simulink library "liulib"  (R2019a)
settings: Solver=ode45  StartTime=0.0  StopTime=10.0  RelTol=1e-3  EnableMultiTasking=on
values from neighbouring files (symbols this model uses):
  ag = NaN(L.ng,1)    [bdet.m]
  D = meqp()    [fbtp.m]
  dr2FA = dr2Fs(1:nA,1)    [asxycs.m]
  drzFA = drzFs(1:nA,1)    [asxycs.m]
  dz = dzxs(is)    [asxycsJac.m]    (also in bintc.m = (z - zx(kz))/dzx)
  dz2FA = dz2Fs(1:nA,1)    [asxycs.m]
  err = [IaeH            ; IoeH               ; IueH               ; DeH               ; FeH            ; BeH               ; BeH               ; BeH               ; CeH               ; CeH               ; CeH               ; VeH                ; VeH                ; VeH               ]    [fbtopt.m]
  FA = Fs(1:nA,1)    [asxycs.m]    (also in bfhelp.m = [-1                        0        0       ])
  FB = [0                         1        1       ]    [bfhelp.m]
  Fx = meqFx(L,Iy,[Ia;Iu])    [bdet.m]    (also in bfhelp.m = zeros(n+2,3); Fx(2:end-1,2) = FN)
  FX = Fs(nA+1:ns,1)    [asxycs.m]
  IpD = LXs.Ip    [fbtinit.m]
  Iy = LXt.Iy    [bdet.m]    (also in fbtinit.m = meqinitIy(L,LXs.t,IpD,bbs,LXs.capaj))
  L = fbtc(P,G)    [fbt.m]    (also in fbtc.m = meqc(P,G); fbte.m = varargout{1})
  nA = numel(rA)    [asxycs.m]
  niter = L.P.itercs    [asxycs.m]
  Opy = logical(Opy)    [bfct.m]    (also in bfdoublet.m = Opy==1 | Opy==2)
  rA = rs(1:nA,1)    [asxycs.m]    (also in fbtptcv.m = (rA1 + 3*rA2)/4)
  rX = rs(nA+1:ns,1)    [asxycs.m]    (also in fbtptcv.m = rzbro(iX,1); fbtxana.m = r0)
  zA = zs(1:nA,1)    [asxycs.m]    (also in fbtptcv.m = (zA1 + 3*zA2)/4)
  zX = zs(nA+1:ns,1)    [asxycs.m]    (also in fbtptcv.m = rzbro(iX,2); fbtxana.m = 0)
undefined symbols (not defined in the file or in its folder): aminor, aq, aW, Bm, bp, bpli2, Brn, Brrn, Brzn, bt, Bzn, Bzrn, Bzzn, delta, deltal, deltau, dzg, epsilon, Ff, Fn, Ft, Ft0, FW, Ie, Ip, iqQ, iTQ, jtorQ, kappa, lB, li, lp, lX, mu, nX, PpQ, PQ, Q0Q, Q1Q, Q2Q, Q3Q, Q4Q, q95, qmin, raQ, raqmin, rB, rbary, rBt, repmat, rgeom, rIp, rIpD, Row, rq, rS, rst, rYD, TQ, TTpQ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
libraries: $bdroot x53, mkllib x48, simulink x7
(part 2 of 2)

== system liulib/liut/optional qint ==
  "LY " : Inport
  Fx : Inport  Port=2
  direct pass : Subsystem  VariantControl=liuINFCTMODEvariant1
  "qint " : Subsystem  VariantControl=liuINFCTMODEvariant2
  " LYo" : Outport

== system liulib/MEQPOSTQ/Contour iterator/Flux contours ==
  zaq : Inport
  rst : Inport  Port=2
  rA : Inport  Port=3
  zA : Inport  Port=4
  FA : Inport  Port=5
  FB : Inport  Port=6
  Fx : Inport  Port=7
  Opy : Inport  Port=8
  IC=1 : UnitDelay  InitialCondition=1  SampleTime=-1  HasFrameUpgradeWarning=on
  Opo : Constant  Value=int8(1)
  RTCI : $bdroot/RTCI  c=L.cdrq  s=L.cdzq  da=L.drx  nr=L.nrx  nz=L.nzx
  Sum : Sum  Inputs=|+-
  Sum1 : Sum  Inputs=|+-
  Sum5 : Sum  Inputs=|+-
  "aq " : Switch  Criteria=u2 ~= 0
  aq0 : Subsystem  TreatAsAtomicUnit=on
  dan : Terminator
  fq : Gain  Gain=L.fq  ParamDataTypeStr=single  OutDataTypeStr=single
  idrx : Gain  Gain=L.idrx  ParamDataTypeStr=single  OutDataTypeStr=single
  idzx : Gain  Gain=L.idzx  ParamDataTypeStr=single  OutDataTypeStr=single
  qaq3 : Sum  Inputs=|++
  rx1 : Constant  Value=L.G.rx(1)  OutDataTypeStr=single
  zx1 : Constant  Value=L.G.zx(1)  OutDataTypeStr=single
  aq : Outport
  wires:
  qaq3/1 -> RTCI/5
  Fx/1 -> RTCI/4
  idzx/1 -> RTCI/3
  idrx/1 -> RTCI/2
  RTCI/2 -> dan/1
  zaq/1 -> "aq "/3
  aq0/1(aq) -> "aq "/1
  "aq "/1 -> RTCI/1
  rA/1 -> Sum/1, aq0/1(rA)
  rx1/1 -> Sum/2
  Sum/1 -> idrx/1
  zA/1 -> Sum1/1, aq0/2(zA)
  zx1/1 -> Sum1/2
  Sum1/1 -> idzx/1
  Sum5/1 -> fq/1
  fq/1 -> qaq3/1
  FB/1 -> Sum5/2, qaq3/2
  FA/1 -> RTCI/7, Sum5/1
  RTCI/1 -> aq/1  "aq"
  Opy/1 -> RTCI/6
  Opo/1 -> RTCI/8
  rst/1 -> IC=1/1
  IC=1/1 -> aq0/Enable, "aq "/2

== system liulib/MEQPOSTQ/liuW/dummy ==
  LY : Inport
  LYo : Outport
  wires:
  LY/1 -> LYo/1

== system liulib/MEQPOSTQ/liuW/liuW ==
  LY : Inport
  Bus Assignment : BusAssignment  AssignedSignals=aW,FW
  Bus Selector : BusSelector  OutputSignals=rst,Fx,Opy,FB,FX,lX,nX
  MATLAB Function : MATLAB Function  TreatAsAtomicUnit=on  mask{nFW=L.P.nFW}
  liuW : Subsystem  VariantControl=liuAWMODEvariant1
  LYo : Outport
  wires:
  Bus Selector/7 -> MATLAB Function/4(nX)  "<nX>"
  Bus Selector/6 -> MATLAB Function/3(lX)  "<lX>"
  Bus Selector/5 -> MATLAB Function/2(FX)  "<FX>"
  Bus Selector/4 -> MATLAB Function/1(FB)  "<FB>"
  Bus Selector/2 -> liuW/2(Fx)  "<Fx>"
  Bus Selector/3 -> liuW/3(Opy)  "<Opy>"
  Bus Selector/1 -> liuW/1(rst)  "<rst>"
  LY/1 -> Bus Selector/1, Bus Assignment/1
  MATLAB Function/1(FW) -> Bus Assignment/3, liuW/4(FW)
  liuW/1(aW) -> Bus Assignment/2
  Bus Assignment/1 -> LYo/1

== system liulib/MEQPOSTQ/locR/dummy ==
  LY : Inport
  "raQ " : Inport  Port=2
  "qQ " : Inport  Port=3
  sq : Inport  Port=4
  Terminator : Terminator
  Terminator1 : Terminator
  Terminator2 : Terminator
  " LYo" : Outport
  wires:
  "raQ "/1 -> Terminator/1
  "qQ "/1 -> Terminator1/1
  sq/1 -> Terminator2/1
  LY/1 -> " LYo"/1

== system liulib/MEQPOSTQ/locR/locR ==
  LY : Inport
  raQ : Inport  Port=2
  qQ : Inport  Port=3
  sq : Inport  Port=4
  Apply sign : Product  Inputs=**
  Bus Assignment : BusAssignment  AssignedSignals=raR
  Constant3 : Constant  Value=L.P.iqR  OutDataTypeStr=single
  Constant4 : Constant  Value=L.raN  OutDataTypeStr=single
  locR : $bdroot/locR  nR=L.nR  naR=L.P.naR
  " LYo" : Outport
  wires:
  Constant4/1 -> locR/4
  qQ/1 -> locR/2
  sq/1 -> Apply sign/2
  Apply sign/1 -> locR/3
  raQ/1 -> locR/1
  Constant3/1 -> Apply sign/1
  locR/1 -> Bus Assignment/2  "raR"
  LY/1 -> Bus Assignment/1
  Bus Assignment/1 -> " LYo"/1

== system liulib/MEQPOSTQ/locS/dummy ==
  "LY " : Inport
  " LYo" : Outport
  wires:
  "LY "/1 -> " LYo"/1

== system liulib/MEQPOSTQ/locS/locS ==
  LY : Inport
  Bus Assignment4 : BusAssignment  AssignedSignals=rS,zS
  Bus Selector : BusSelector  OutputSignals=aq,raQ,rA,zA
  Constant1 : Constant  Value=L.P.raS  OutDataTypeStr=single
  Constant2 : Constant  Value=L.raN  OutDataTypeStr=single
  Matrix Concatenate : Concatenate  Mode=Multidimensional array  ConcatenateDimension=2
  RTCI1 : $bdroot/RTCI1  SFunctionModules=''
  RTCI2 : $bdroot/RTCI1  SFunctionModules=''
  crq : Constant  Value=L.crq  OutDataTypeStr=single
  czq : Constant  Value=L.czq  OutDataTypeStr=single
  locS : $bdroot/locS  SFunctionModules=''
  row of zeros : Constant  Value=zeros(L.noq,1)  OutDataTypeStr=Inherit: Inherit via back propagation
  LYo : Outport
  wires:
  Bus Selector/4 -> RTCI2/3  "<zA>"
  Bus Assignment4/1 -> LYo/1
  LY/1 -> Bus Selector/1, Bus Assignment4/1
  locS/1 -> RTCI1/1, RTCI2/1
  Matrix Concatenate/1 -> locS/1
  Bus Selector/2 -> locS/2  "<raQ>"
  Constant1/1 -> locS/3
  czq/1 -> RTCI2/2
  crq/1 -> RTCI1/2
  Bus Selector/3 -> RTCI1/3  "<rA>"
  RTCI2/1 -> Bus Assignment4/3
  RTCI1/1 -> Bus Assignment4/2
  Constant2/1 -> locS/4
  row of zeros/1 -> Matrix Concatenate/1
  Bus Selector/1 -> Matrix Concatenate/2  "<aq>"

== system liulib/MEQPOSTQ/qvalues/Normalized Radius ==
  aq : Inport
  Constant : Constant  Value=0  OutDataTypeStr=single
  Normalise : Product  Inputs=*/
  Outboard radius : Selector  NumberOfDimensions=2  InputPortWidth=3  IndexOptions=Index vector (dialog),Select all  Indices=find(L.crq==1),L.npq  OutputSizes=1,1
  Permute Dimensions : PermuteDimensions
  Reshape : Reshape
  Reshape1 : Reshape
  Vector Concatenate : Concatenate
  end value : Selector  InputPortWidth=L.npq  IndexOptions=Index vector (dialog)  Indices=L.npq  OutputSizes=1
  raQ : Outport
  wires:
  Outboard radius/1 -> Reshape1/1
  Reshape1/1 -> end value/1, Normalise/1
  Constant/1 -> Vector Concatenate/1
  aq/1 -> Outboard radius/1
  Normalise/1 -> Vector Concatenate/2
  end value/1 -> Normalise/2
  Reshape/1 -> raQ/1
  Permute Dimensions/1 -> Reshape/1
  Vector Concatenate/1 -> Permute Dimensions/1

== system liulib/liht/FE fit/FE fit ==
  Yd : Inport
  Ie : Inport  Port=2
  Ip_in : Inport  Port=3
  sIp : Inport  Port=4
  FE : $bdroot/FE  SystemSampleTime=-1  Latency=0  AutoFrameSizeCalculation=off
  Iph : mkllib/A*u  A=L.Iph
  Iph_D : mkllib/A*u  A=[L.Iph_t;L.Iph_b]
  Iprh : mkllib/A*u  A=L.Iprh
  Iprh_D : mkllib/A*u  A=[L.Iprh_t;L.Iprh_b]
  Ipzh : mkllib/A*u  A=L.Ipzh
  Ipzh_D : mkllib/A*u  A=[L.Ipzh_t;L.Ipzh_b]
  Subsystem1 : Subsystem
  Variant Source : VariantSource
  Variant Source1 : VariantSource
  Variant Source2 : VariantSource
  Je : Outport
  IpD : Outport  Port=2
  rIpD : Outport  Port=3
  zIpD : Outport  Port=4
  Ip : Outport  Port=5
  rIp : Outport  Port=6
  zIp : Outport  Port=7
  rYD : Outport  Port=8
  zYD : Outport  Port=9
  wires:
  Variant Source2/1 -> zIpD/1, Subsystem1/3(zIpD)
  Variant Source1/1 -> Subsystem1/2(rIpD), rIpD/1  "rIpD"
  Variant Source/1 -> IpD/1, Subsystem1/1(IpD)
  Subsystem1/1(rYD) -> rYD/1  "rYD"
  Subsystem1/2(zYD) -> zYD/1  "zYD"
  FE/2 -> Je/1
  sIp/1 -> FE/4
  Yd/1 -> FE/1
  Ip_in/1 -> FE/3
  Ie/1 -> FE/2
  Iprh_D/1 -> Variant Source1/1  "rIpD"
  FE/1 -> Iph_D/1, Ipzh/1, Iprh/1, Iph/1, Ipzh_D/1, Iprh_D/1
  Iph_D/1 -> Variant Source/1  "IpD"
  Ipzh_D/1 -> Variant Source2/1  "zIpD"
  Iprh/1 -> rIp/1, Variant Source1/2  "rIp"
  Iph/1 -> Ip/1, Variant Source/2  "Ip"
  Ipzh/1 -> zIp/1, Variant Source2/2  "zIp"

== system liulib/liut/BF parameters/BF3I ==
  BF3I parameters : Subsystem
  Bus Creator : BusCreator  Inputs=4
  bfp : Outport
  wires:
  BF3I parameters/2(IgNg) -> Bus Creator/2
  BF3I parameters/4(fTg) -> Bus Creator/4
  BF3I parameters/3(fPg) -> Bus Creator/3
  Bus Creator/1 -> bfp/1
  BF3I parameters/1(gNg) -> Bus Creator/1

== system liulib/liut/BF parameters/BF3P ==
  Constant : Constant  Value=L.P.bfp
  bfp : Outport
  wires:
  Constant/1 -> bfp/1

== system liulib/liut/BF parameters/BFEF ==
  Constant : Constant  Value=L.P.bfp
  bfp : Outport
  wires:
  Constant/1 -> bfp/1

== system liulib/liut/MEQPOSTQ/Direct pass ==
  "LY " : Inport
  "sIp " : Inport  Port=2
  Terminator : Terminator
  " LYo" : Outport
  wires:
  "LY "/1 -> " LYo"/1
  "sIp "/1 -> Terminator/1

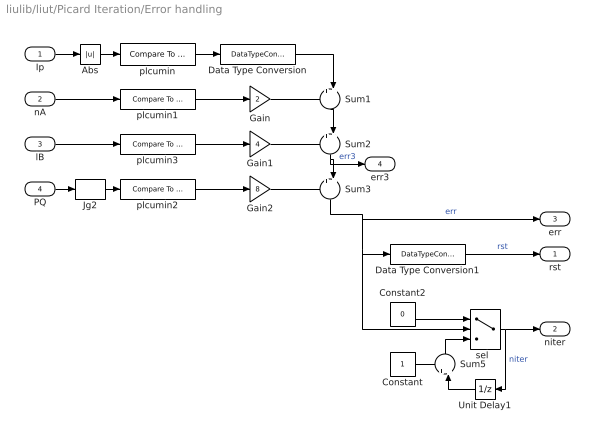
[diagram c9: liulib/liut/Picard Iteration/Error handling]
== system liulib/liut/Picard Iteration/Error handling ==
  Ip : Inport
  nA : Inport  Port=2
  lB : Inport  Port=3
  PQ : Inport  Port=4
  Abs : Abs
  Constant : Constant  VectorParams1D=off  OutDataTypeStr=int32
  Constant2 : Constant  Value=0  VectorParams1D=off  OutDataTypeStr=int32
  Data Type Conversion : DataTypeConversion  OutDataTypeStr=int32
  Data Type Conversion1 : DataTypeConversion  OutDataTypeStr=boolean
  Gain : Gain  Gain=2  OutDataTypeStr=int32
  Gain1 : Gain  Gain=4  OutDataTypeStr=int32
  Gain2 : Gain  Gain=8  OutDataTypeStr=int32
  Jg2 : Selector  IndexMode=Zero-based  IndexOptions=Index vector (dialog)  Indices=0  OutputSizes=1
  Sum{1..3,5} (4 alike) : Sum  Inputs=++|
  Unit Delay1 : UnitDelay  InitialCondition=int32(0)  SampleTime=-1  HasFrameUpgradeWarning=on
  plcumin : simulink/Logic and Bit Operations/Compare To Constant  relop=<  const=L.P.Ipmin  OutDataTypeStr=uint8
  plcumin1 : simulink/Logic and Bit Operations/Compare To Constant  relop===  const=0  OutDataTypeStr=uint8
  plcumin2 : simulink/Logic and Bit Operations/Compare To Constant  relop=<  const=0  OutDataTypeStr=uint8
  plcumin3 : simulink/Logic and Bit Operations/Compare To Constant  relop===  const=0  OutDataTypeStr=uint8
  "sel  " : Switch  Criteria=u2 ~= 0  OutDataTypeStr=int32
  rst : Outport
  niter : Outport  Port=2
  err : Outport  Port=3
  err3 : Outport  Port=4
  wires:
  plcumin2/1 -> Gain2/1
  nA/1 -> plcumin1/1
  Jg2/1 -> plcumin2/1
  PQ/1 -> Jg2/1
  Data Type Conversion1/1 -> rst/1  "rst"
  Ip/1 -> Abs/1
  Abs/1 -> plcumin/1
  "sel  "/1 -> niter/1, Unit Delay1/1  "niter"
  Sum5/1 -> "sel  "/3
  Constant/1 -> Sum5/1
  lB/1 -> plcumin3/1
  plcumin3/1 -> Gain1/1
  Unit Delay1/1 -> Sum5/2
  Constant2/1 -> "sel  "/1
  plcumin1/1 -> Gain/1
  plcumin/1 -> Data Type Conversion/1
  Gain1/1 -> Sum2/1
  Gain2/1 -> Sum3/1
  Sum3/1 -> "sel  "/2, Data Type Conversion1/1, err/1  "err"
  Gain/1 -> Sum1/1
  Data Type Conversion/1 -> Sum1/2
  Sum1/1 -> Sum2/2
  Sum2/1 -> err3/1, Sum3/2  "err3"

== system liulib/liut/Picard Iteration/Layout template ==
  u : Inport
  y : Outport
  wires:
  u/1 -> y/1

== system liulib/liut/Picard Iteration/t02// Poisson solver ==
  rst : Inport
  Yd : Inport  Port=2
  Ie : Inport  Port=3
  Ip : Inport  Port=4
  sIp : Inport  Port=5
  zJy : Inport  Port=6
  zJe : Inport  Port=7
  zdz : Inport  Port=8
  *idzx : Gain  Gain=single(L.idzx)
  Constant2 : Constant  Value=0  OutDataTypeStr=single
  Fb : Switch  Criteria=u2 ~= 0
  Fb BF : Subsystem  TreatAsAtomicUnit=on
  Fb FE : Subsystem  TreatAsAtomicUnit=on
  GSZR : $bdroot/GSZR  cx=L.cx  cq=L.cq  cr=L.cr  cs=L.cs  ci=L.ci  co=L.co
  Je : Switch  Criteria=u2 ~= 0
  Jw : $bdroot/ASGN  iu=L.kyw-1
  "Jy " : Switch  Criteria=u2 ~= 0
  KYWMODE : VariantSource
  Logical Operator : Logic  Operator=NOT  IconShape=distinctive  AllPortsSameDT=off  OutDataTypeStr=boolean
  Mbe : mkllib/A*u  A=L.Mbe
  Sum3 : Sum
  Tww : mkllib/A*u  A=single(L.Tww)
  dz : Switch  Criteria=u2 ~= 0
  kew : Selector  IndexMode=Zero-based  IndexOptions=Index vector (dialog)  Indices=L.kew-1  OutputSizes=1
  Jy : Outport
  Fx : Outport  Port=2
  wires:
  Yd/1 -> Fb FE/1(Yd)
  GSZR/1 -> Fx/1  "Fx"
  zdz/1 -> dz/3, Fb BF/3(dz)  "zdz"
  zJe/1 -> Fb BF/2(Je)  "zJe"
  kew/1 -> Tww/1
  rst/1 -> Fb FE/Enable, Fb/2, Je/2, dz/2, Logical Operator/1, "Jy "/2
  Logical Operator/1 -> Fb BF/Enable
  zJy/1 -> Fb BF/1(Jy)  "zJy"
  Mbe/1 -> Sum3/2
  Je/1 -> Mbe/1, kew/1
  Fb/1 -> Sum3/1  "Fb"
  "Jy "/1 -> Jw/1, KYWMODE/1, Jy/1  "Jy"
  Fb FE/3(Je) -> Je/1
  Fb FE/2(Fb) -> Fb/1
  Fb BF/2(Fb) -> Fb/3
  Tww/1 -> Jw/2
  Fb FE/1(Jy) -> "Jy "/1
  dz/1 -> *idzx/1
  Constant2/1 -> dz/1
  Ie/1 -> Fb FE/2(Ie)
  Ip/1 -> Fb FE/3(Ip)
  sIp/1 -> Fb FE/4(sIp)
  Fb BF/3(=Je) -> Je/3
  Fb BF/1(=Jy) -> "Jy "/3
  Jw/1 -> KYWMODE/2
  KYWMODE/1 -> GSZR/1
  Sum3/1 -> GSZR/2
  *idzx/1 -> GSZR/3

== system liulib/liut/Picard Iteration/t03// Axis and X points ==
  Fx : Inport
  FN : Inport  Port=2
  ASXY : $bdroot/ASXY  rx=L.G.rx  zx=L.G.zx  dr=L.drx  dz=L.dzx  idr=L.idrx  idz=L.idzx  Oasx=L.Oasx  daxm=L.P.dasm
  Terminator{,1..3} (4 alike) : Terminator
  Vector Concatenate : Concatenate  NumInputs=3
  rA : Outport
  zA : Outport  Port=2
  FA : Outport  Port=3
  d2FA : Outport  Port=4
  nA : Outport  Port=5
  rX : Outport  Port=6
  zX : Outport  Port=7
  FX : Outport  Port=8
  nX : Outport  Port=9
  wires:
  ASXY/8 -> rX/1  "rX"
  ASXY/5 -> Vector Concatenate/2
  ASXY/10 -> FX/1  "FX"
  ASXY/9 -> zX/1  "zX"
  ASXY/4 -> Vector Concatenate/1
  Fx/1 -> ASXY/1
  ASXY/1 -> rA/1  "rA"
  ASXY/6 -> Vector Concatenate/3
  ASXY/15 -> Terminator3/1  "stat"
  ASXY/11 -> Terminator/1  "dr2FX"
  ASXY/3 -> FA/1  "FA"
  ASXY/13 -> Terminator2/1  "drzFX"
  FN/1 -> ASXY/2
  ASXY/14 -> nX/1  "nX"
  ASXY/2 -> zA/1  "zA"
  ASXY/12 -> Terminator1/1  "dz2FX"
  ASXY/7 -> nA/1  "nA"
  Vector Concatenate/1 -> d2FA/1  "d2FA"

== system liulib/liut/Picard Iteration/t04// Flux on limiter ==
  note: % Exclude limiter points with wrong sign of derivative away from axis
  note: % Exclude candidate limiter points outside x-point polygon
  rA : Inport
  zA : Inport  Port=2
  rX : Inport  Port=3
  zX : Inport  Port=4
  nX : Inport  Port=5
  Fx : Inport  Port=6
  FN : Inport  Port=7
  Constant : Constant  Value=L.G.rl  OutDataTypeStr=single
  Constant1 : Constant  Value=L.G.zl  OutDataTypeStr=single
  FL4P : $bdroot/FL4P  kl=int32(L.kxl-1)  cl=L.clx  nz=L.nzx
  Sum : Sum  Inputs=-+|
  Sum1 : Sum  Inputs=-+|
  Switch : Switch  Criteria=u2 ~= 0
  Switch1 : Switch  Criteria=u2 > Threshold  ZeroCross=off
  dAFl : Subsystem
  dAfl*FN : Product
  l in OX : $bdroot/l in OX1  a=0
  Fl : Outport
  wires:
  nX/1 -> l in OX/5
  l in OX/1 -> Switch/2
  FL4P/1 -> Switch/1
  rX/1 -> Sum/1, l in OX/1
  zX/1 -> Sum1/1, l in OX/2
  rA/1 -> dAFl/2(rA), Sum/2
  Sum/1 -> l in OX/3
  zA/1 -> dAFl/5(zA), Sum1/2
  Sum1/1 -> l in OX/4
  Fx/1 -> FL4P/1
  Constant/1 -> l in OX/6, dAFl/3(rl)
  Constant1/1 -> l in OX/7, dAFl/6(zl)
  Switch1/1 -> Fl/1
  dAFl/1(dAFl) -> dAfl*FN/1
  dAfl*FN/1 -> Switch1/2
  Switch/1 -> Switch1/3
  FN/1 -> Switch/3, Switch1/1, dAfl*FN/2, FL4P/2
  FL4P/2 -> dAFl/1(drFl)
  FL4P/3 -> dAFl/4(dzFl)

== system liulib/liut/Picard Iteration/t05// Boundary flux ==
  rA : Inport
  zA : Inport  Port=2
  Fl : Inport  Port=3
  FX : Inport  Port=4
  rX : Inport  Port=5
  zX : Inport  Port=6
  nX : Inport  Port=7
  FN : Inport  Port=8
  Sum : Sum  Inputs=+-
  Sum1 : Sum  Inputs=+-
  Switch : Switch  Criteria=u2 ~= 0
  l in OX1 : $bdroot/l in OX1  a=0
  t05/ Boundary flux : $bdroot/FBND  rl=L.G.rl  zl=L.G.zl
  FB : Outport
  rB : Outport  Port=2
  zB : Outport  Port=3
  lB : Outport  Port=4
  lX : Outport  Port=5
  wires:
  Fl/1 -> t05/ Boundary flux/1
  t05/ Boundary flux/1 -> FB/1  "FB"
  t05/ Boundary flux/2 -> rB/1  "rB"
  t05/ Boundary flux/3 -> zB/1  "zB"
  t05/ Boundary flux/4 -> lB/1  "lB"
  t05/ Boundary flux/5 -> lX/1  "lX"
  FX/1 -> Switch/1
  rX/1 -> Sum/2, l in OX1/1, l in OX1/6, t05/ Boundary flux/3
  zX/1 -> l in OX1/2, l in OX1/7, t05/ Boundary flux/4, Sum1/2
  nX/1 -> l in OX1/5, t05/ Boundary flux/5
  FN/1 -> Switch/3, t05/ Boundary flux/6
  rA/1 -> Sum/1
  Sum/1 -> l in OX1/3
  zA/1 -> Sum1/1
  Sum1/1 -> l in OX1/4
  l in OX1/1 -> Switch/2
  Switch/1 -> t05/ Boundary flux/2

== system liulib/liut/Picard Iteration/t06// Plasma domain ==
  rA : Inport
  zA : Inport  Port=2
  rX : Inport  Port=3
  zX : Inport  Port=4
  nX : Inport  Port=5
  Fx : Inport  Port=6
  FB : Inport  Port=7
  Ip : Inport  Port=8
  Constant : Constant  Value=L.ry  OutDataTypeStr=Inherit: Inherit via back propagation
  Constant1 : Constant  Value=L.zy  OutDataTypeStr=Inherit: Inherit via back propagation
  Data Type Conversion : DataTypeConversion  OutDataTypeStr=int8
  OXy : $bdroot/BAVX2  a=0
  PDOM : $bdroot/PDOM
  Sum : Sum  Inputs=-+|
  Sum1 : Sum  Inputs=-+|
  Opy : Outport
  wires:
  Fx/1 -> PDOM/1
  FB/1 -> PDOM/2
  Ip/1 -> PDOM/3
  nX/1 -> OXy/5
  OXy/1 -> PDOM/4
  Constant1/1 -> OXy/7
  Constant/1 -> OXy/6
  rX/1 -> Sum/1, OXy/1
  zX/1 -> Sum1/1, OXy/2
  rA/1 -> Sum/2
  Sum/1 -> OXy/3
  Sum1/1 -> OXy/4
  zA/1 -> Sum1/2
  PDOM/1 -> Data Type Conversion/1  "Opy"
  Data Type Conversion/1 -> Opy/1

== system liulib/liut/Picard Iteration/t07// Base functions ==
  Fx : Inport
  Opy : Inport  Port=2
  FA : Inport  Port=3
  FB : Inport  Port=4
  bfp : Inport  Port=5
  err : Inport  Port=6
  bf3i : Subsystem  VariantControl=liuBFCTMODEvariant2
  bf3p : Subsystem  VariantControl=liuBFCTMODEvariant1
  bfef : Subsystem  VariantControl=liuBFCTMODEvariant3
  Tyg : Outport
  Tpg : Outport  Port=2
  ITpg : Outport  Port=3
  fPg : Outport  Port=4
  fTg : Outport  Port=5

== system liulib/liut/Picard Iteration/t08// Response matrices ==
  Tyg : Inport
  Jy : Inport  Port=2
  Tpg : Inport  Port=3
  ITpg : Inport  Port=4
  fTg : Inport  Port=5
  rBt : Inport  Port=6
  Add : Sum
  Constant1 : Constant  Value=L.Mty  OutDataTypeStr=single
  Gain : Gain  Gain=repmat(L.Wr,1,L.nj)
  Product : Product  Inputs=3
  Product1 : Product
  Reshape : Reshape  OutputDimensionality=Row vector (2-D)
  Wi j : Concatenate  Mode=Multidimensional array  ConcatenateDimension=2
  Wp : Gain  Gain=L.Wp
  Wriz : Concatenate  Mode=Multidimensional array
  Wt : Gain  Gain=L.Wt
  "[0;0]" : Constant  Value=[0;0]  OutDataTypeStr=single
  "[Mry*Tyg Mdzry*Jy]" : $bdroot/RESP  A=L.Mry  B=L.Mdzry*L.P.fdz  nr=L.nr  ng=L.ng
  mu0/2pi : Constant  Value=single(2e-7)  OutDataTypeStr=single
  v*U : mkllib/v*U  alpha=1  order=102  transA=112  incx=1  beta=0  incy=1
  Wrj : Outport
  Wij : Outport  Port=2
  Mrj : Outport  Port=3
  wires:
  Gain/1 -> Wrj/1
  ITpg/1 -> Product/1
  Tpg/1 -> Wp/1
  Wp/1 -> Wriz/2
  Wt/1 -> Wriz/1
  Wriz/1 -> Wi j/1
  "[0;0]"/1 -> Wi j/2
  Wi j/1 -> Wij/1
  "[Mry*Tyg Mdzry*Jy]"/1 -> Gain/1, Mrj/1
  fTg/1 -> Product/2
  Jy/1 -> "[Mry*Tyg Mdzry*Jy]"/2
  Tyg/1 -> v*U/1, "[Mry*Tyg Mdzry*Jy]"/1
  mu0/2pi/1 -> Product/3
  v*U/1 -> Product1/1
  rBt/1 -> Product1/2
  Product1/1 -> Reshape/1
  Add/1 -> Wt/1
  Product/1 -> Add/2
  Constant1/1 -> v*U/2
  Reshape/1 -> Add/1

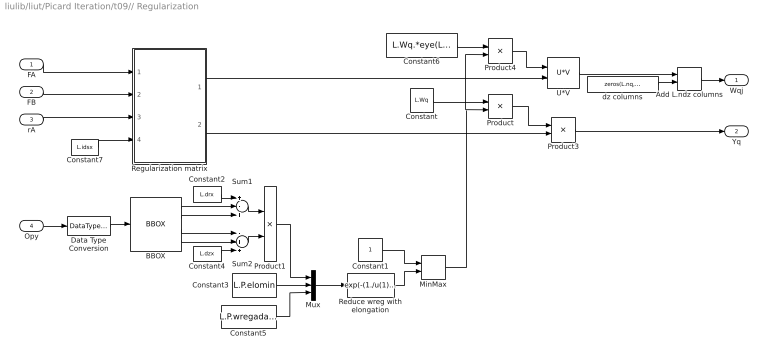
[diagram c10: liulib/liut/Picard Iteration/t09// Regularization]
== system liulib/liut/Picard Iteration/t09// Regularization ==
  FA : Inport
  FB : Inport  Port=2
  rA : Inport  Port=3
  Opy : Inport  Port=4
  Add L.ndz columns : Concatenate  Mode=Multidimensional array  ConcatenateDimension=2
  BBOX : $bdroot/BBOX  z=L.zy  r=L.ry
  Constant : Constant  Value=L.Wq  OutDataTypeStr=single
  Constant1 : Constant  OutDataTypeStr=single
  Constant2 : Constant  Value=L.drx  OutDataTypeStr=single
  Constant3 : Constant  Value=L.P.elomin  OutDataTypeStr=single
  Constant4 : Constant  Value=L.dzx  OutDataTypeStr=single
  Constant5 : Constant  Value=L.P.wregadapt  OutDataTypeStr=single
  Constant6 : Constant  Value=L.Wq.*eye(L.nq)  OutDataTypeStr=single
  Constant7 : Constant  Value=L.idsx  OutDataTypeStr=single
  Data Type Conversion : DataTypeConversion  OutDataTypeStr=boolean
  MinMax : MinMax  Inputs=2
  Mux : Mux  Inputs=3
  Product : Product
  Product1 : Product  Inputs=*/
  Product3 : Product
  Product4 : Product
  Reduce wreg with elongation : Fcn  Expr=exp(-(1./u(1)-u(2))*u(3))
  Regularization matrix : Subsystem  Variant=on  VariantControl=Variant1
  Sum1 : Sum  Inputs=+-+
  Sum2 : Sum  Inputs=-++
  U*V : mkllib/U*V  a=1
  dz columns : Constant  Value=zeros(L.nq,L.ndz)  OutDataTypeStr=single
  Wqj : Outport
  Yq : Outport  Port=2
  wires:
  FA/1 -> Regularization matrix/1("FA ")
  FB/1 -> Regularization matrix/2("FB ")
  rA/1 -> Regularization matrix/3("rA ")
  Constant7/1 -> Regularization matrix/4("ids ")
  BBOX/1 -> Sum1/2
  Sum2/1 -> Product1/2
  Constant2/1 -> Sum1/1
  Sum1/1 -> Product1/1
  BBOX/4 -> Sum2/2
  BBOX/2 -> Sum1/3
  Constant4/1 -> Sum2/3
  BBOX/3 -> Sum2/1
  Reduce wreg with elongation/1 -> MinMax/2
  Constant/1 -> Product/1
  Product3/1 -> Yq/1
  U*V/1 -> Add L.ndz columns/1
  Add L.ndz columns/1 -> Wqj/1
  Constant1/1 -> MinMax/1
  MinMax/1 -> Product4/2, Product/2
  Mux/1 -> Reduce wreg with elongation/1
  Constant6/1 -> Product4/1
  Product/1 -> Product3/1
  Regularization matrix/2(" Xq") -> Product3/2
  Product4/1 -> U*V/1
  Regularization matrix/1(" Qqg") -> U*V/2
  Product1/1 -> Mux/1
  Constant3/1 -> Mux/2
  Constant5/1 -> Mux/3
  Opy/1 -> Data Type Conversion/1
  Data Type Conversion/1 -> BBOX/1
  dz columns/1 -> Add L.ndz columns/2

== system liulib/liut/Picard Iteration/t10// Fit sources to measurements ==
  Wrj : Inport
  Wij : Inport  Port=2
  Wqj : Inport  Port=3
  Yr : Inport  Port=4
  Yi : Inport  Port=5
  Yq : Inport  Port=6
  Yd : Inport  Port=7
  Ie : Inport  Port=8
  Double precision : Subsystem  VariantControl=liuBSLVMODEvariant2
  Single precision : Subsystem  VariantControl=liuBSLVMODEvariant1
  ag : Outport
  dzg : Outport  Port=2
  Je : Outport  Port=3

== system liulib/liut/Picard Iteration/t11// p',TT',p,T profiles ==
  ag : Inport
  FA : Inport  Port=2
  FB : Inport  Port=3
  fPg : Inport  Port=4
  fTg : Inport  Port=5
  rBt : Inport  Port=6
  Small diamagnetism approximation : Subsystem
  p',TT',p,hqT profiles : Subsystem  VariantControl=BFCTMODE==1
  PpQ : Outport
  TTpQ : Outport  Port=2
  PQ : Outport  Port=3
  hqTQ : Outport  Port=4
  TQ : Outport  Port=5
  iTQ : Outport  Port=6
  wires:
  fPg/1 -> p',TT',p,hqT profiles/4(fPg)
  ag/1 -> p',TT',p,hqT profiles/1(ag)
  Small diamagnetism approximation/2(iT) -> iTQ/1  "iTQ"
  Small diamagnetism approximation/1(T) -> TQ/1  "TQ"
  rBt/1 -> Small diamagnetism approximation/2(rBt)
  p',TT',p,hqT profiles/4(hqTQ) -> Small diamagnetism approximation/1(hqT), hqTQ/1
  FA/1 -> p',TT',p,hqT profiles/2(FA)
  p',TT',p,hqT profiles/1(PpQ) -> PpQ/1
  p',TT',p,hqT profiles/2(TTpQ) -> TTpQ/1
  p',TT',p,hqT profiles/3(PQ) -> PQ/1
  FB/1 -> p',TT',p,hqT profiles/3(FB)
  fTg/1 -> p',TT',p,hqT profiles/5(fTg)

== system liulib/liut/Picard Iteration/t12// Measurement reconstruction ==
  Mrj : Inport
  ag : Inport  Port=2
  dzg : Inport  Port=3
  Ie : Inport  Port=4
  1/fdz : Gain  Gain=1/L.P.fdz
  Add : Sum
  Gain : Gain  Gain=L.Mre  Multiplication=Matrix(K*u) (u vector)
  Selector : Selector  IndexOptions=Index vector (dialog)  Indices=1:L.G.nf  OutputSizes=1
  Selector1 : Selector  IndexOptions=Index vector (dialog)  Indices=L.G.nf + (1:L.G.nm)  OutputSizes=1
  U*v : mkllib/U*v  a=1
  Vector Concatenate : Concatenate
  Bm : Outport
  Ff : Outport  Port=2
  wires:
  Selector/1 -> Ff/1  "Ff"
  Selector1/1 -> Bm/1  "Bm"
  Add/1 -> Selector/1, Selector1/1
  Gain/1 -> Add/2
  Ie/1 -> Gain/1
  U*v/1 -> Add/1
  Mrj/1 -> U*v/1
  Vector Concatenate/1 -> U*v/2  "aj"
  dzg/1 -> 1/fdz/1
  ag/1 -> Vector Concatenate/1
  1/fdz/1 -> Vector Concatenate/2

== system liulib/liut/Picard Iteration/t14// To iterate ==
  Tyg : Inport
  ag : Inport  Port=2
  Je : Inport  Port=3
  dz : Inport  Port=4
  rst : Inport  Port=5
  Jx : mkllib/U*v  a=1
  Unit Delay : UnitDelay  InitialCondition=1  SampleTime=-1  HasFrameUpgradeWarning=on
  Unit Delay1 : UnitDelay  SampleTime=-1  HasFrameUpgradeWarning=on
  Unit Delay2 : UnitDelay  SampleTime=-1  HasFrameUpgradeWarning=on
  Unit Delay4 : UnitDelay  SampleTime=-1  HasFrameUpgradeWarning=on
  Iy : Outport
  zJy : Outport  Port=2
  zJe : Outport  Port=3
  zdz : Outport  Port=4
  zrst : Outport  Port=5
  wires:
  rst/1 -> Unit Delay/1
  Unit Delay/1 -> zrst/1
  Je/1 -> Unit Delay2/1
  Unit Delay2/1 -> zJe/1
  ag/1 -> Jx/2
  dz/1 -> Unit Delay1/1
  Tyg/1 -> Jx/1
  Jx/1 -> Unit Delay4/1, Iy/1  "Iy"
  Unit Delay4/1 -> zJy/1
  Unit Delay1/1 -> zdz/1

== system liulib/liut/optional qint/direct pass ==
  LY : Inport
  Fx : Inport  Port=2
  Terminator : Terminator
  LYo : Outport
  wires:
  Fx/1 -> Terminator/1
  LY/1 -> LYo/1

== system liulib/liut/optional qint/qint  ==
  note: Loop voltage calculation at interpolation points by Finite Differences
  LY : Inport
  Fx : Inport  Port=2
  Add : Sum  Inputs=+-
  Bus Assignment3 : BusAssignment  AssignedSignals=Fn,Brn,Bzn,Brrn,Brzn,Bzrn,Bzzn,Un
  Constant1 : Constant  Value=single(L.P.rn)
  Constant2 : Constant  Value=single(L.P.zn)
  Gain : Gain  Gain=single(1/L.dt)
  Memory : Memory
  QINT : $bdroot/QINT  rx=L.rx  zx=L.zx  inM=L.inM
  Switch : Switch  Criteria=u2 ~= 0
  LYo : Outport
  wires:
  Gain/1 -> Switch/1
  Switch/1 -> Bus Assignment3/9
  Add/1 -> Gain/1
  QINT/1 -> Bus Assignment3/2, Add/1, Memory/1
  Memory/1 -> Add/2, Switch/2, Switch/3
  Fx/1 -> QINT/1
  QINT/7 -> Bus Assignment3/8
  QINT/6 -> Bus Assignment3/7
  QINT/5 -> Bus Assignment3/6
  QINT/4 -> Bus Assignment3/5
  QINT/3 -> Bus Assignment3/4
  QINT/2 -> Bus Assignment3/3
  Constant2/1 -> QINT/3
  Constant1/1 -> QINT/2
  LY/1 -> Bus Assignment3/1
  Bus Assignment3/1 -> LYo/1

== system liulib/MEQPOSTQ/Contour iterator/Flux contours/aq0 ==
  rA : Inport
  zA : Inport  Port=2
  rst : EnablePort
  Sum{,1..3} (4 alike) : Sum  Inputs=|+-
  a1 : MinMax  Inputs=4
  pq0 : Gain  Gain=L.pinit*repmat(L.pq,L.noq,1)
  rx1 : Constant  Value=L.G.rx(1)  OutDataTypeStr=single
  rx9 : Constant  Value=L.G.rx(end)  OutDataTypeStr=single
  zx1 : Constant  Value=L.G.zx(1)  OutDataTypeStr=single
  zx9 : Constant  Value=L.G.zx(end)  OutDataTypeStr=single
  aq : Outport
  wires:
  a1/1 -> pq0/1
  Sum2/1 -> a1/4
  Sum3/1 -> a1/3
  Sum/1 -> a1/2
  Sum1/1 -> a1/1
  zx9/1 -> Sum3/1
  zA/1 -> Sum2/1, Sum3/2
  zx1/1 -> Sum2/2
  rx9/1 -> Sum1/1
  rA/1 -> Sum1/2, Sum/1
  rx1/1 -> Sum/2
  pq0/1 -> aq/1

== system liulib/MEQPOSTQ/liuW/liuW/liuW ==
  rst : Inport
  Fx : Inport  Port=2
  Opy : Inport  Port=3
  FW : Inport  Port=4
  For Iterator : ForIterator  IterationLimit=L.P.iterq  ShowIterationPort=off
  Unit Delay : UnitDelay  SampleTime=-1  HasFrameUpgradeWarning=on
  liuW : $bdroot/liuW  SystemSampleTime=-1  Latency=0  AutoFrameSizeCalculation=off
  aW : Outport
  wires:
  Opy/1 -> liuW/5
  Fx/1 -> liuW/4
  FW/1 -> liuW/3
  rst/1 -> liuW/2
  Unit Delay/1 -> liuW/1
  liuW/1 -> aW/1, Unit Delay/1

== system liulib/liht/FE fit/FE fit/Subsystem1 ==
  IpD : Inport
  rIpD : Inport  Port=2
  zIpD : Inport  Port=3
  Constant : Constant  Value=0  OutDataTypeStr=Inherit: Inherit via back propagation
  Divide2 : Product  Inputs=*/
  Divide3 : Product  Inputs=*/
  Switch2 : Switch  Criteria=u2 ~= 0
  Switch3 : Switch  Criteria=u2 ~= 0
  rYD : Outport
  zYD : Outport  Port=2
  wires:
  Switch3/1 -> zYD/1
  rIpD/1 -> Divide2/1
  Divide3/1 -> Switch3/1
  Switch2/1 -> rYD/1
  Constant/1 -> Switch3/3, Switch2/3
  zIpD/1 -> Divide3/1
  IpD/1 -> Divide2/2, Switch2/2, Switch3/2, Divide3/2
  Divide2/1 -> Switch2/1

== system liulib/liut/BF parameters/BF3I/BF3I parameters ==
  Constant : Constant  Value=L.P.bfp.gNg  VectorParams1D=off  OutDataTypeStr=single
  Constant1 : Constant  Value=L.P.bfp.IgNg  VectorParams1D=off  OutDataTypeStr=single
  Constant2 : Constant  Value=L.P.bfp.fPg  OutDataTypeStr=single
  Constant3 : Constant  Value=L.P.bfp.fTg  OutDataTypeStr=single
  gNg : Outport
  IgNg : Outport  Port=2
  fPg : Outport  Port=3
  fTg : Outport  Port=4
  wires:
  Constant/1 -> gNg/1
  Constant3/1 -> fTg/1
  Constant2/1 -> fPg/1
  Constant1/1 -> IgNg/1

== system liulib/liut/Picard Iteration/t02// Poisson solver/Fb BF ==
  Jy : Inport
  Je : Inport  Port=2
  dz : Inport  Port=3
  ~rst : EnablePort
  Add : Sum  Inputs=+-
  Constant : Constant  Value=0  OutDataTypeStr=single
  Constant1 : Constant  Value=zeros(1,(L.nzy+L.nry)*2+4)  OutDataTypeStr=single
  Divide : Product  Inputs=**
  GSZR BC=0 : Subsystem  TreatAsAtomicUnit=on
  NFDB : $bdroot/NFDB  nz=L.nzx  nr=L.nrx
  Tbc : mkllib/A*u  A=single(L.Tbc)
  dzMbe : mkllib/A*u  A=single(L.dzMbe)
  =Jy : Outport
  Fb : Outport  Port=2
  =Je : Outport  Port=3
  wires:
  Jy/1 -> GSZR BC=0/1(Iy), =Jy/1
  dzMbe/1 -> Add/2
  Add/1 -> Fb/1
  Divide/1 -> dzMbe/1
  dz/1 -> Divide/2
  Je/1 -> =Je/1, Divide/1
  Tbc/1 -> Add/1
  NFDB/1 -> Tbc/1
  Constant1/1 -> GSZR BC=0/2(Fb)
  Constant/1 -> GSZR BC=0/3(dz)
  GSZR BC=0/1(Fx) -> NFDB/1

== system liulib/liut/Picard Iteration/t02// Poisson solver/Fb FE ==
  Yd : Inport
  Ie : Inport  Port=2
  Ip : Inport  Port=3
  sIp : Inport  Port=4
  rst : EnablePort
  FE : $bdroot/FE  SystemSampleTime=-1
  Mbh* : mkllib/A*u  A=L.Mbh
  Tyh* : mkllib/A*u  A=L.Tyh
  Jy : Outport
  Fb : Outport  Port=2
  Je : Outport  Port=3
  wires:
  Mbh*/1 -> Fb/1
  Tyh*/1 -> Jy/1
  Yd/1 -> FE/1
  FE/2 -> Je/1
  Ie/1 -> FE/2
  Ip/1 -> FE/3
  sIp/1 -> FE/4
  FE/1 -> Mbh*/1, Tyh*/1

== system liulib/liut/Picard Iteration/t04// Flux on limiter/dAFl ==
  note: % Flux derivative away from axis dAFl = (drFl.*(rA-rl) + dzFl.*(zA-zl));
  drFl : Inport
  rA : Inport  Port=2
  rl : Inport  Port=3
  dzFl : Inport  Port=4
  zA : Inport  Port=5
  zl : Inport  Port=6
  Product : Product
  Product1 : Product
  Sum : Sum  Inputs=|+-
  Sum1 : Sum  Inputs=|+-
  Sum2 : Sum  Inputs=|++
  dAFl : Outport  VectorParamsAs1DForOutWhenUnconnected=on
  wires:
  drFl/1 -> Product1/1
  rA/1 -> Sum/1
  rl/1 -> Sum/2
  zA/1 -> Sum1/1
  zl/1 -> Sum1/2
  Sum/1 -> Product1/2
  Sum1/1 -> Product/2
  dzFl/1 -> Product/1
  Product1/1 -> Sum2/1
  Product/1 -> Sum2/2
  Sum2/1 -> dAFl/1

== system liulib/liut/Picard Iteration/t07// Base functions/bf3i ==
  Fx : Inport
  Opy : Inport  Port=2
  FA : Inport  Port=3
  FB : Inport  Port=4
  bfp : Inport  Port=5
  err : Inport  Port=6
  BF3I1 : $bdroot/BF3I1  r=L.ry  ir=L.iry  nz=L.nzy  nr=L.nry
  Demux : Demux  BusSelectionMode=on
  Tyg : Outport
  Tpg : Outport  Port=2
  ITpg : Outport  Port=3
  fPg : Outport  Port=4
  fTg : Outport  Port=5
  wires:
  Fx/1 -> BF3I1/1
  Opy/1 -> BF3I1/2
  FA/1 -> BF3I1/3
  FB/1 -> BF3I1/4
  BF3I1/1 -> Tyg/1
  BF3I1/2 -> Tpg/1
  BF3I1/3 -> ITpg/1
  Demux/1 -> BF3I1/5
  Demux/2 -> BF3I1/6
  Demux/3 -> BF3I1/7, fPg/1
  bfp/1 -> Demux/1
  Demux/4 -> fTg/1, BF3I1/8
  err/1 -> BF3I1/9

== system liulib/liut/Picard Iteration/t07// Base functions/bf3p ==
  Fx : Inport
  Opy : Inport  Port=2
  FA : Inport  Port=3
  FB : Inport  Port=4
  bfp : Inport  Port=5
  err : Inport  Port=6
  BF3P1 : $bdroot/BF3P1  ry=L.ry  iry=L.iry  nzy=L.nzy  nry=L.nry
  Constant : Constant  Value=[1 0 0]  VectorParams1D=off  OutDataTypeStr=single
  Constant1 : Constant  Value=[0 1 1]  VectorParams1D=off  OutDataTypeStr=single
  Constant2 : Constant  Value=false
  Terminator : Terminator
  Tyg : Outport
  Tpg : Outport  Port=2
  ITpg : Outport  Port=3
  fPg : Outport  Port=4
  fTg : Outport  Port=5
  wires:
  err/1 -> BF3P1/6
  FB/1 -> BF3P1/4
  FA/1 -> BF3P1/3
  Fx/1 -> BF3P1/1
  BF3P1/1 -> Tyg/1
  BF3P1/3 -> ITpg/1
  BF3P1/2 -> Tpg/1
  Constant2/1 -> BF3P1/5
  Opy/1 -> BF3P1/2
  bfp/1 -> Terminator/1
  Constant/1 -> fPg/1
  Constant1/1 -> fTg/1

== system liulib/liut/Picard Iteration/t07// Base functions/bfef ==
  Fx : Inport
  Opy : Inport  Port=2
  FA : Inport  Port=3
  FB : Inport  Port=4
  bfp : Inport  Port=5
  err : Inport  Port=6
  BFEF1 : $bdroot/BFEF1  ry=L.ry  iry=L.iry  nzy=L.nzy  nry=L.nry  nP=L.P.bfp(1)  nT=L.P.bfp(2)
  Constant1 : Constant  Value=L.fTg  OutDataTypeStr=single
  Constant2 : Constant  Value=L.fPg  OutDataTypeStr=single
  Terminator : Terminator
  Tyg : Outport
  Tpg : Outport  Port=2
  ITpg : Outport  Port=3
  fPg : Outport  Port=4
  fTg : Outport  Port=5
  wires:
  Fx/1 -> BFEF1/1
  Opy/1 -> BFEF1/2
  FA/1 -> BFEF1/3
  FB/1 -> BFEF1/4
  err/1 -> BFEF1/5
  BFEF1/3 -> ITpg/1
  BFEF1/2 -> Tpg/1
  BFEF1/1 -> Tyg/1
  Constant2/1 -> fPg/1
  Constant1/1 -> fTg/1
  bfp/1 -> Terminator/1

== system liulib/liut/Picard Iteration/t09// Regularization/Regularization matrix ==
  "FA " : Inport
  "FB " : Inport  Port=2
  "rA " : Inport  Port=3
  "ids " : Inport  Port=4
  bf3i : Subsystem  VariantControl=liuBFCTMODEvariant2
  bf3p : Subsystem  VariantControl=liuBFCTMODEvariant1
  bfef : Subsystem  VariantControl=liuBFCTMODEvariant3
  " Qqg" : Outport
  " Xq" : Outport  Port=2

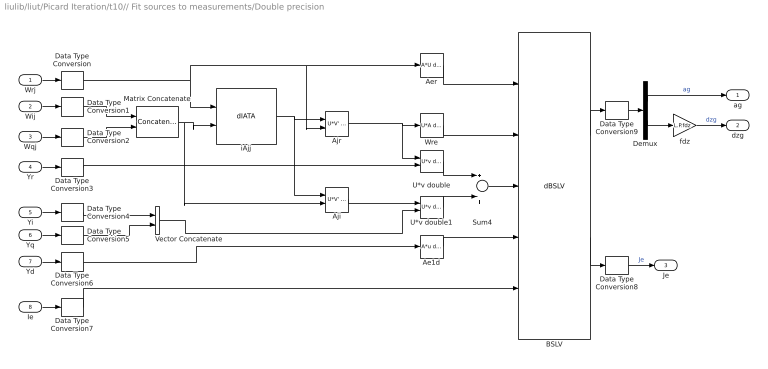
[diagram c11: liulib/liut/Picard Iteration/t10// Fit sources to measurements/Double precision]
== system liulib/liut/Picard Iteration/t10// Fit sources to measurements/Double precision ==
  Wrj : Inport
  Wij : Inport  Port=2
  Wqj : Inport  Port=3
  Yr : Inport  Port=4
  Yi : Inport  Port=5
  Yq : Inport  Port=6
  Yd : Inport  Port=7
  Ie : Inport  Port=8
  Ae1d : mkllib/A*u double  A=L.Ae1d
  Aer : mkllib/A*U double  A=L.Aer
  Aji : mkllib/U*V' double  a=1
  Ajr : mkllib/U*V' double  a=1
  BSLV : $bdroot/dBSLV  niter=L.P.iters
  Data Type Conversion{,1..7} (8 alike) : DataTypeConversion  OutDataTypeStr=double
  Data Type Conversion8 : DataTypeConversion  OutDataTypeStr=single
  Data Type Conversion9 : DataTypeConversion  OutDataTypeStr=single
  Demux : Demux  Outputs=[L.ng L.ndz]
  Matrix Concatenate : Concatenate  Mode=Multidimensional array
  Sum4 : Sum  Inputs=+|+
  U*v double : mkllib/U*v double  a=1
  U*v double1 : mkllib/U*v double  a=1
  Vector Concatenate : Concatenate
  Wre : mkllib/U*A double  A=L.Wre
  fdz : Gain  Gain=L.P.fdz
  iAjj : $bdroot/dIATA  SFunctionModules=''
  ag : Outport
  dzg : Outport  Port=2
  Je : Outport  Port=3
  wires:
  Wij/1 -> Data Type Conversion1/1
  Wrj/1 -> Data Type Conversion/1
  Yd/1 -> Data Type Conversion6/1
  Yi/1 -> Data Type Conversion4/1
  Ajr/1 -> U*v double/1, Wre/1
  BSLV/2 -> Data Type Conversion8/1
  Ae1d/1 -> BSLV/4
  Wre/1 -> BSLV/2
  Aer/1 -> BSLV/1
  Ie/1 -> Data Type Conversion7/1
  Demux/2 -> fdz/1
  Demux/1 -> ag/1  "ag"
  BSLV/1 -> Data Type Conversion9/1
  Yr/1 -> Data Type Conversion3/1
  Aji/1 -> U*v double1/1
  U*v double/1 -> Sum4/1
  U*v double1/1 -> Sum4/2
  Sum4/1 -> BSLV/3
  iAjj/1 -> Ajr/1, Aji/1
  fdz/1 -> dzg/1  "dzg"
  Data Type Conversion/1 -> iAjj/1, Ajr/2, Aer/1
  Data Type Conversion3/1 -> U*v double/2
  Data Type Conversion6/1 -> Ae1d/1
  Data Type Conversion7/1 -> BSLV/5
  Data Type Conversion8/1 -> Je/1  "Je"
  Data Type Conversion9/1 -> Demux/1
  Yq/1 -> Data Type Conversion5/1
  Wqj/1 -> Data Type Conversion2/1
  Data Type Conversion1/1 -> Matrix Concatenate/1
  Data Type Conversion2/1 -> Matrix Concatenate/2
  Matrix Concatenate/1 -> Aji/2, iAjj/2
  Data Type Conversion4/1 -> Vector Concatenate/1
  Data Type Conversion5/1 -> Vector Concatenate/2
  Vector Concatenate/1 -> U*v double1/2

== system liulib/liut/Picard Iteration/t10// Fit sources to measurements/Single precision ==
  Wrj : Inport
  Wij : Inport  Port=2
  Wqj : Inport  Port=3
  Yr : Inport  Port=4
  Yi : Inport  Port=5
  Yq : Inport  Port=6
  Yd : Inport  Port=7
  Ie : Inport  Port=8
  Ae1d : mkllib/A*u  A=L.Ae1d
  Aer : mkllib/A*U  A=L.Aer
  Aji : mkllib/U*V'  a=1
  Ajr : mkllib/U*V'  a=1
  BSLV : $bdroot/sBSLV  niter=L.P.iters
  Demux : Demux  Outputs=[L.ng L.ndz]
  Matrix Concatenate : Concatenate  Mode=Multidimensional array
  Sum4 : Sum  Inputs=+|+
  Vector Concatenate : Concatenate
  Wre : mkllib/U*A  A=L.Wre
  fdz : Gain  Gain=L.P.fdz
  iAjj : $bdroot/sIATA  SFunctionModules=''
  xg1 : mkllib/U*v  a=1
  xg2 : mkllib/U*v  a=1
  ag : Outport
  dzg : Outport  Port=2
  Je : Outport  Port=3
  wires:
  Wrj/1 -> iAjj/1, Aer/1, Ajr/2
  Yd/1 -> Ae1d/1
  Ajr/1 -> xg1/1, Wre/1
  BSLV/2 -> Je/1  "Je"
  Ae1d/1 -> BSLV/4
  Wre/1 -> BSLV/2
  Aer/1 -> BSLV/1
  Ie/1 -> BSLV/5
  Demux/2 -> fdz/1
  Demux/1 -> ag/1  "ag"
  BSLV/1 -> Demux/1
  Yr/1 -> xg1/2
  Aji/1 -> xg2/1
  xg1/1 -> Sum4/1
  xg2/1 -> Sum4/2
  Sum4/1 -> BSLV/3
  iAjj/1 -> Aji/1, Ajr/1
  fdz/1 -> dzg/1  "dz"
  Matrix Concatenate/1 -> Aji/2, iAjj/2
  Wij/1 -> Matrix Concatenate/1
  Wqj/1 -> Matrix Concatenate/2
  Yi/1 -> Vector Concatenate/1
  Yq/1 -> Vector Concatenate/2
  Vector Concatenate/1 -> xg2/2

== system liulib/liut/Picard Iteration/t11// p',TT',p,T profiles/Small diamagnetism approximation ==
  hqT : Inport
  rBt : Inport  Port=2
  Constant : Constant  OutDataTypeStr=single
  Constant1 : Constant  Value=2  OutDataTypeStr=single
  Sum1 : Sum
  Sum2 : Sum  Inputs=-+
  ahqTg1 : Product
  ahqTg2 : Product
  ahqTg3 : Product
  irBt : Product  Inputs=/*
  T : Outport
  iT : Outport  Port=2
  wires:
  ahqTg2/1 -> Sum2/1
  Constant1/1 -> Sum2/2
  irBt/1 -> ahqTg2/2, ahqTg3/2, ahqTg1/2
  Sum1/1 -> ahqTg2/1, T/1
  Constant/1 -> irBt/2
  ahqTg1/1 -> Sum1/1
  rBt/1 -> irBt/1, Sum1/2
  hqT/1 -> ahqTg1/1
  ahqTg3/1 -> iT/1
  Sum2/1 -> ahqTg3/1

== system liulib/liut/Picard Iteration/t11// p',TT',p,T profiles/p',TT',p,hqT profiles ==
  ag : Inport
  FA : Inport  Port=2
  FB : Inport  Port=3
  fPg : Inport  Port=4
  fTg : Inport  Port=5
  Base functions on rho grid Coefficients for source terms : Subsystem  Variant=on
  Constant : Constant  Value=L.TQg  VectorParams1D=off  OutDataTypeStr=single
  Constant1 : Constant  Value=L.ITQg  VectorParams1D=off  OutDataTypeStr=single
  smvunv{,1..3} (4 alike) : mkllib/U*v  a=1
  PpQ : Outport
  TTpQ : Outport  Port=2
  PQ : Outport  Port=3
  hqTQ : Outport  Port=4
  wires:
  smvunv2/1 -> PQ/1  "PQ"
  smvunv/1 -> PpQ/1  "PpQ"
  Constant1/1 -> smvunv3/1, smvunv2/1
  FA/1 -> Base functions on rho grid Coefficients for source terms/2(FA)
  FB/1 -> Base functions on rho grid Coefficients for source terms/3(FB)
  ag/1 -> Base functions on rho grid Coefficients for source terms/1(ag)
  Base functions on rho grid Coefficients for source terms/1(aPpg) -> smvunv/2
  Base functions on rho grid Coefficients for source terms/2(aTTpg) -> smvunv1/2
  Base functions on rho grid Coefficients for source terms/3(aPg) -> smvunv2/2
  Base functions on rho grid Coefficients for source terms/4(ahqTg) -> smvunv3/2
  fPg/1 -> Base functions on rho grid Coefficients for source terms/4(fPg)
  fTg/1 -> Base functions on rho grid Coefficients for source terms/5(fTg)
  smvunv3/1 -> hqTQ/1  "hqTQ"
  smvunv1/1 -> TTpQ/1  "TTpQ"
  Constant/1 -> smvunv1/1, smvunv/1

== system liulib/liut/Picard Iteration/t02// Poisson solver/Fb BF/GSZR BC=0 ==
  note: This subsystem is mecessary to allow treating this as an atomic subsystem. Otherwise we would get improper real-time behaviour
  Iy : Inport
  Fb : Inport  Port=2
  dz : Inport  Port=3
  GSZR : $bdroot/GSZR  cx=L.cx  cq=L.cq  cr=L.cr  cs=L.cs  ci=L.ci  co=L.co
  Fx : Outport
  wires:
  dz/1 -> GSZR/3
  Iy/1 -> GSZR/1
  Fb/1 -> GSZR/2
  GSZR/1 -> Fx/1

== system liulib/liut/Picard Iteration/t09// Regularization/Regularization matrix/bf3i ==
  "FA " : Inport
  "FB " : Inport  Port=2
  "rA " : Inport  Port=3
  "ids " : Inport  Port=4
  BF3I6 : $bdroot/BF3I6  SFunctionModules=''
  Terminator{,1..3} (4 alike) : Terminator
  " Qqg" : Outport
  " Xq" : Outport  Port=2
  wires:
  BF3I6/1 -> " Qqg"/1
  BF3I6/2 -> " Xq"/1
  "FA "/1 -> Terminator/1
  "FB "/1 -> Terminator1/1
  "rA "/1 -> Terminator2/1
  "ids "/1 -> Terminator3/1

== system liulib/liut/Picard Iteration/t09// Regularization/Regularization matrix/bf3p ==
  "FA " : Inport
  "FB " : Inport  Port=2
  "rA " : Inport  Port=3
  "ids " : Inport  Port=4
  BF3P6 : $bdroot/BF3P6  SFunctionModules=''
  Divide : Product  Inputs=/
  " Qqg" : Outport
  " Xq" : Outport  Port=2
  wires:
  "FA "/1 -> BF3P6/1
  "FB "/1 -> BF3P6/2
  Divide/1 -> BF3P6/3
  "ids "/1 -> BF3P6/4
  BF3P6/2 -> " Xq"/1
  BF3P6/1 -> " Qqg"/1
  "rA "/1 -> Divide/1

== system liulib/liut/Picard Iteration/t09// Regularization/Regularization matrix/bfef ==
  "FA " : Inport
  "FB " : Inport  Port=2
  "rA " : Inport  Port=3
  "ids " : Inport  Port=4
  BFEF6 : $bdroot/BFEF6  nP=L.P.bfp(1)  nT=L.P.bfp(2)  nq=L.nq
  Divide : Product  Inputs=/
  " Qqg" : Outport
  " Xq" : Outport  Port=2
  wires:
  BFEF6/1 -> " Qqg"/1
  BFEF6/2 -> " Xq"/1
  "FA "/1 -> BFEF6/1
  "FB "/1 -> BFEF6/2
  "rA "/1 -> Divide/1, BFEF6/3
  Divide/1 -> BFEF6/4
  "ids "/1 -> BFEF6/5

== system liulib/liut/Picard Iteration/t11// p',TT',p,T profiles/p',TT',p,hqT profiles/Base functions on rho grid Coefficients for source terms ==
  ag : Inport
  FA : Inport  Port=2
  FB : Inport  Port=3
  fPg : Inport  Port=4
  fTg : Inport  Port=5
  bf3i : Subsystem  VariantControl=liuBFCTMODEvariant2
  bf3p : Subsystem  VariantControl=liuBFCTMODEvariant1
  bfef : Subsystem  VariantControl=liuBFCTMODEvariant3
  aPpg : Outport
  aTTpg : Outport  Port=2
  aPg : Outport  Port=3
  ahqTg : Outport  Port=4

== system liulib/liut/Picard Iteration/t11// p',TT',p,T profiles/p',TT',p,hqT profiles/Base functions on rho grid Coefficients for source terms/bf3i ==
  ag : Inport
  FA : Inport  Port=2
  FB : Inport  Port=3
  fPg : Inport  Port=4
  fTg : Inport  Port=5
  BF3I3 : $bdroot/BF3I3  idsx=L.idsx
  aPpg : Outport
  aTTpg : Outport  Port=2
  aPg : Outport  Port=3
  ahqTg : Outport  Port=4
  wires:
  fPg/1 -> BF3I3/4
  fTg/1 -> BF3I3/5
  ag/1 -> BF3I3/1
  FA/1 -> BF3I3/2
  FB/1 -> BF3I3/3
  BF3I3/1 -> aPpg/1
  BF3I3/2 -> aTTpg/1
  BF3I3/3 -> aPg/1
  BF3I3/4 -> ahqTg/1

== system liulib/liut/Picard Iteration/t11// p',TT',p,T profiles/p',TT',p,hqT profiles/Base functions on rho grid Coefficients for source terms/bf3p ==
  ag : Inport
  FA : Inport  Port=2
  FB : Inport  Port=3
  fPg : Inport  Port=4
  fTg : Inport  Port=5
  BF3P3 : $bdroot/BF3P3  idsx=L.idsx
  Terminator1 : Terminator
  Terminator2 : Terminator
  aPpg : Outport
  aTTpg : Outport  Port=2
  aPg : Outport  Port=3
  ahqTg : Outport  Port=4
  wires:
  BF3P3/4 -> ahqTg/1
  BF3P3/3 -> aPg/1
  BF3P3/2 -> aTTpg/1
  BF3P3/1 -> aPpg/1
  FB/1 -> BF3P3/3
  FA/1 -> BF3P3/2
  ag/1 -> BF3P3/1
  fTg/1 -> Terminator1/1
  fPg/1 -> Terminator2/1

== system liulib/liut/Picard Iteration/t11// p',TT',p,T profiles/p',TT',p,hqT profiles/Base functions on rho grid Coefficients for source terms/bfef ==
  ag : Inport
  FA : Inport  Port=2
  FB : Inport  Port=3
  fPg : Inport  Port=4
  fTg : Inport  Port=5
  BFEF3 : $bdroot/BFEF3  ids=L.idsx  nP=L.P.bfp(1)  nT=L.P.bfp(2)
  Terminator : Terminator
  Terminator1 : Terminator
  aPpg : Outport
  aTTpg : Outport  Port=2
  aPg : Outport  Port=3
  ahqTg : Outport  Port=4
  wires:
  ag/1 -> BFEF3/1
  FA/1 -> BFEF3/2
  FB/1 -> BFEF3/3
  BFEF3/1 -> aPpg/1
  BFEF3/2 -> aTTpg/1
  BFEF3/3 -> aPg/1
  BFEF3/4 -> ahqTg/1
  fPg/1 -> Terminator/1
  fTg/1 -> Terminator1/1

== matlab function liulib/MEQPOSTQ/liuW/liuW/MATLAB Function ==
function FW = meqFW(FB,FX,lX,nX,nFW)

FW = meqFW(FB,FX(1:nX),lX,nX,nFW);

end
